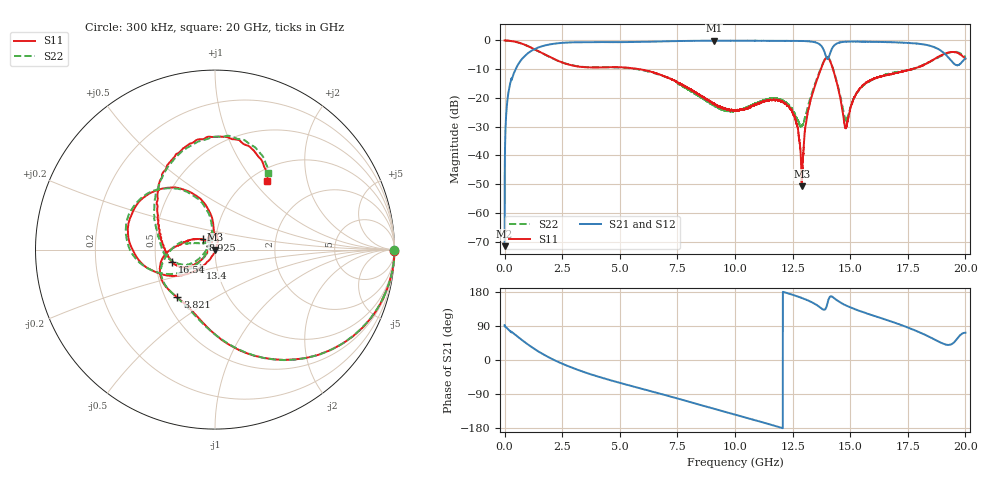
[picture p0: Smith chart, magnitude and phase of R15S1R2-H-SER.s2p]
!{R15S1R2}
!Johanson Technology Inc.
!www.johansontechnology.com
!Test Board Conditions:
!Substrate Type  RO4350B
!Substrate Thickness  20 mil
!Substrate Dk  3.66
!TL Type: GCPW
!TL Trace Width  34 mil
!TL Gap  10 mil
!Electrode orientation  Horizontal
!DUT TOPOLOGY	SERIES
!Mounting Pad LxW  26x52 mil
! Created Sat Feb  6 12:12:10 2021
# hz S ma R 50
! 2 Port Network Data from SP1.SP block
! freq  magS11  angS11  magS21  angS21  magS12  angS12  magS22  angS22
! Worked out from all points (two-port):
!   20001 points, 300 kHz to 20 GHz, reference 50 ohm
!   highest |S21| = -0.07 dB at 9.084 GHz (marker M1); lowest = -71.6 dB at 300 kHz (marker M2)
!   |S21| within 3 dB of the highest: 1.286 GHz to 13.83 GHz (12.55 GHz wide, 166 % of centre); 14.2 GHz to 18.84 GHz (4.647 GHz wide, 28.1 % of centre)
!   lowest |S11| = -50.8 dB at 12.9 GHz (marker M3), VSWR 1.01, Z = 50.3 - j0.0975 ohm
!   |S11| at or under -10 dB: 5.833 GHz to 13.73 GHz (7.894 GHz wide, 80.7 % of centre); 14.25 GHz to 17.69 GHz (3.433 GHz wide, 21.5 % of centre); 17.68736 GHz to 17.69394 GHz (6.586 MHz wide, 0.0372 % of centre)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
!   |S22| runs from -30.0 to 0.0 dB; largest |S21 - S12| = 0.016
!   S11 on the Smith chart (normalised r, x): 300 kHz: open; 3.821 GHz: 0.58, -0.35; 8.925 GHz: 0.87, +0.10; 13.4 GHz: 0.83, -0.17; 16.54 GHz: 0.61, -0.09; 20 GHz: 1.19, +1.17
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300000  1 -0.3  0.0002624 92.0  0.0002345 87.9  0.9977 -0.2
1.363e8  0.994 -7.6  0.1017 82.3  0.1023 82.2  0.9944 -7.4
5.243e8  0.9374 -26.3  0.3446 63.5  0.3457 63.5  0.9363 -26.2
1.8653e9  0.5381 -81.2  0.8382 8.8  0.8396 8.8  0.5371 -81.0
3.3343e9  0.3469 -118.7  0.9337 -29.3  0.9338 -29.4  0.3485 -119.7
3.8213e9  0.3392 -128.3  0.937 -39.3  0.9373 -39.3  0.3404 -129.8
6.6673e9  0.2607 -177.9  0.9585 -87.5  0.9598 -87.5  0.257 -176.8
8.9253e9  0.08647 139.4  0.9902 -125.9  0.9906 -125.9  0.07969 154.4
9.0843e9  0.08052 137.5  0.9916 -128.6  0.9891 -128.7  0.07513 150.7
1.00003e10  0.06022 133.1  0.9896 -144.1  0.9899 -144.1  0.06011 124.0
1.21423e10  0.0809 83.8  0.9828 178.9  0.9822 178.8  0.08606 100.6
1.26313e10  0.04087 70.5  0.9819 169.4  0.9813 169.4  0.04949 113.1
1.28993e10  0.002885 -19.7  0.9779 163.6  0.9782 163.7  0.03313 163.3
1.33343e10  0.1082 -125.6  0.9528 152.4  0.9545 152.4  0.12 -141.0
1.33953e10  0.1308 -129.4  0.9439 150.4  0.9472 150.5  0.1419 -141.5
1.40563e10  0.4931 143.9  0.4973 159.3  0.4969 158.7  0.5023 145.6
1.48193e10  0.0301 162.1  0.9538 143.9  0.9518 144.1  0.04048 151.4
1.54483e10  0.1498 -145.0  0.9569 128.7  0.9561 128.6  0.1471 -148.9
1.65403e10  0.249 -163.9  0.9398 106.5  0.9304 106.4  0.2545 -167.4
1.66673e10  0.2528 -167.3  0.936 103.8  0.9246 103.8  0.2637 -169.3
1.87823e10  0.5112 125.2  0.7238 50.4  0.7247 50.5  0.4959 126.9
2e10  0.4778 52.8  0.4896 71.9  0.4852 72.4  0.5186 55.1
